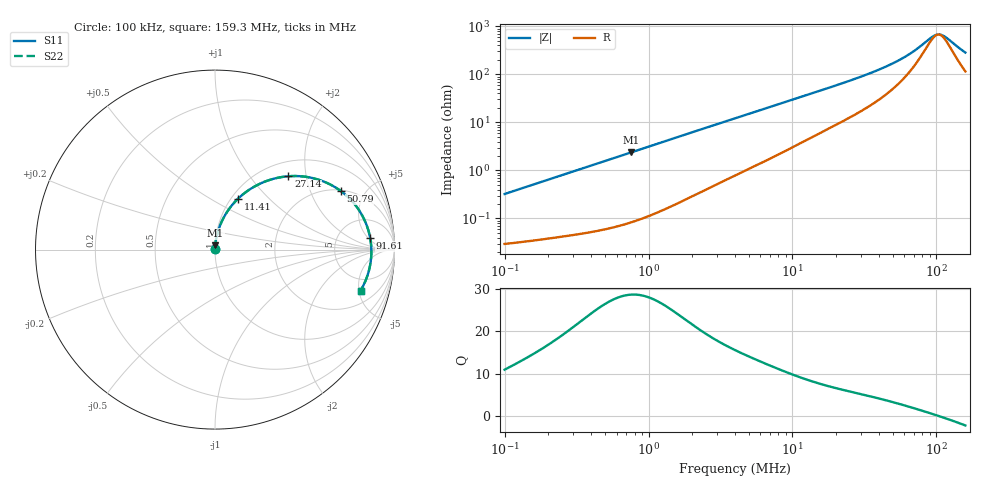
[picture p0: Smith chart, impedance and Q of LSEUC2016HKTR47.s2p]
! LSEUC2016HKTR47  S-PARAMETER MODEL  ( General Type )
! Model Generated by TAIYO YUDEN Corporation (http://www.ty-top.com)
! Version 1.0
! TAIYO YUDEN Control No. 220210
! Copyright(c) 2022 TAIYO YUDEN CO.,LTD. All Rights Reserved.
! Product Description (link to TY-COMPAS)
! https://ds.yuden.co.jp/TYCOMPAS/or/detail?pn=LSEUC2016HKTR47M&u=M
! Products Name : Inductors
! Characteristics :
!  Inductance : 0.47 uH , SRF(min) : -Hz , DC Resistance(max) : 0.028 Ohm
!  Rated Current : Saturation :4900 mA , Temp Rise : 4200 mA (40 degC)
!  Case Size : 2.0 x 1.6 / 0.079 x 0.063 [mm/inch] , Thickness : 0.8 / 0.031 [mm/inch]
!  (Conditions: Temperature = 25 degC , DC Bias Current/Voltage = 0A / 0V)
! External Node Assignments :
!  1  o---GGG---o  2
! GND o---------o GND
! Frequency Range : 0.1MHz  -  159.254811MHz  [ 402 STEP ]
# MHz S RI R 50
! Freq[MHz].  S11 Real  S11 Imag  S21 Real  S21 Imag  S12 Real  S12 Imag  S22 Real  S22 Imag
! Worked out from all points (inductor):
!   401 points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, 100 kHz to 159.3 MHz, reference 50 ohm
!   read as one part in series: L = 510 nH near 103.8 kHz
!   highest Q = 28.6 at 759.6 kHz (marker M1), where L = 498 nH
!   self-resonance near 103.4 MHz
!   S11 on the Smith chart (normalised r, x): 100 kHz: 1.00, +0.01; 11.41 MHz: 1.07, +0.67; 27.14 MHz: 1.29, +1.58; 50.79 MHz: 2.04, +3.32; 91.61 MHz: 11, +6; 159.3 MHz: 3.30, -5.19
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0.1  0.000305 0.00322  0.9997 -0.00322  0.9997 -0.00322  0.000305 0.00322
0.343835  0.000599 0.0108  0.9994 -0.0108  0.9994 -0.0108  0.000599 0.0108
0.759583  0.00139 0.0237  0.9986 -0.0237  0.9986 -0.0237  0.00139 0.0237
1.182227  0.00272 0.0367  0.9973 -0.0367  0.9973 -0.0367  0.00272 0.0367
2.295564  0.00843 0.07  0.9916 -0.07  0.9916 -0.07  0.00843 0.07
4.064915  0.0226 0.1197  0.9774 -0.1197  0.9774 -0.1197  0.0226 0.1197
7.198031  0.0598 0.1982  0.9402 -0.1982  0.9402 -0.1982  0.0598 0.1982
11.41155  0.127 0.2824  0.873 -0.2824  0.873 -0.2824  0.127 0.2824
13.72135  0.1684 0.3178  0.8316 -0.3178  0.8316 -0.3178  0.1684 0.3178
19.12014  0.2681 0.3749  0.7319 -0.3749  0.7319 -0.3749  0.2681 0.3749
27.13878  0.4086 0.4087  0.5914 -0.4087  0.5914 -0.4087  0.4086 0.4087
35.78235  0.5379 0.3999  0.4621 -0.3999  0.4621 -0.3999  0.5379 0.3999
47.17884  0.6678 0.3485  0.3322 -0.3485  0.3322 -0.3485  0.6678 0.3485
50.78883  0.6999 0.3272  0.3001 -0.3272  0.3001 -0.3272  0.6999 0.3272
58.85862  0.7583 0.2755  0.2417 -0.2755  0.2417 -0.2755  0.7583 0.2755
68.21061  0.8066 0.2131  0.1934 -0.2131  0.1934 -0.2131  0.8066 0.2131
91.60847  0.8644 0.0655  0.1356 -0.0655  0.1356 -0.0655  0.8644 0.0655
100.4527  0.8705 0.0157  0.1295 -0.0157  0.1295 -0.0157  0.8705 0.0157
110.1509  0.8706 -0.0347  0.1294 0.0347  0.1294 0.0347  0.8706 -0.0347
118.5793  0.8663 -0.075  0.1337 0.075  0.1337 0.075  0.8663 -0.075
147.9352  0.8304 -0.192  0.1696 0.192  0.1696 0.192  0.8304 -0.192
159.2548  0.8109 -0.2284  0.1891 0.2284  0.1891 0.2284  0.8109 -0.2284
